FUNCTION_BLOCK FB_DO_IED_LD1_LLN0_Mod EXTENDS FB_AcsiCommonControllableDataClass
VAR_INPUT
	stVal: FB_AcsiDATypeMod := (fc:=ACSI_FC_ST, TrgOp:=ACSI_TrgOp_dchg, bLinkResult:=THIS^.AddDataToContainer(ipData:=stVal));
	q: FB_AcsiDATypeQuality := (fc:=ACSI_FC_ST, TrgOp:=ACSI_TrgOp_qchg, bLinkResult:=THIS^.AddDataToContainer(ipData:=q));
	t: FB_AcsiDATypeTimeStamp := (fc:=ACSI_FC_ST, bLinkResult:=THIS^.AddDataToContainer(ipData:=t));
	stSeld: FB_AcsiBATypeBOOLEAN := (fc:=ACSI_FC_ST, TrgOp:=ACSI_TrgOp_dchg, bLinkResult:=THIS^.AddDataToContainer(ipData:=stSeld));
	ctlModel: FB_AcsiDATypeCtlModels := (fc:=ACSI_FC_CF, TrgOp:=ACSI_TrgOp_dchg, eValue:=E_AcsiCtlModels.DirectWithEnhancedSecurity, bLinkResult:=THIS^.AddDataToContainer(ipData:=ctlModel));
	Oper: FB_AcsiCDC_Oper_ENUMERATED := (fc:=ACSI_FC_CO, bLinkResult:=THIS^.AddDataToContainer(ipData:=Oper));
	fbControl: FB_DirectControl := (ipCtrl:=THIS^.AddServerJob(ipEvent:=fbControl, ipCompletion:=fbControl), eType:=E_AcsiCDCType.ENC, ipBehVal:=fbIED.IEDLD1.XCBR1.Beh.stVal);
END_VAR
VAR
END_VAR

END_FUNCTION_BLOCK
